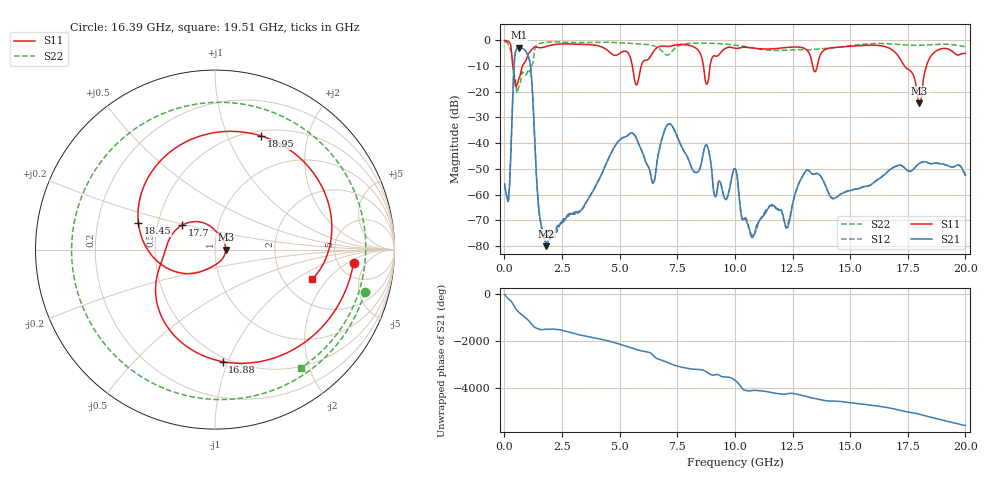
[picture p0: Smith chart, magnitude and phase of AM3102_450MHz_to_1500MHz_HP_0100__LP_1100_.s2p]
!Agilent Technologies,E8364B,MY43040894,A.07.50.67
!Agilent E8364B: A.07.50.67
!Date: Thursday, January 11, 2018 05:38:16
!Correction: S11(Full 2 Port(1,2))
!S21(Full 2 Port(1,2))
!S12(Full 2 Port(1,2))
!S22(Full 2 Port(1,2))
!S2P File: Measurements: S11, S21, S12, S22:
# Hz S  dB  R 50
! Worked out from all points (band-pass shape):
!   1601 points, 10 MHz to 20 GHz, reference 50 ohm
!   highest |S21| = -2.88 dB at 634.7 MHz (marker M1); lowest = -80.1 dB at 1.822 GHz (marker M2)
!   |S21| within 3 dB of the highest: 459.8 MHz to 1.021 GHz (560.8 MHz wide, 75.8 % of centre)
!   lowest |S11| = -24.5 dB at 18 GHz (marker M3), VSWR 1.13, Z = 56.4 + j0.00754 ohm
!   |S11| at or under -10 dB: 366.2 MHz to 781.8 MHz (415.5 MHz wide, 72.4 % of centre); 5.551 GHz to 5.938 GHz (387.2 MHz wide, 6.74 % of centre); 17.36 GHz to 18.31 GHz (951.1 MHz wide, 5.33 % of centre)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
!   |S22| runs from -20.5 to -0.5 dB; largest |S21 - S12| = 0.0025
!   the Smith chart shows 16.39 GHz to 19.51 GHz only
!   S11 on the Smith chart (normalised r, x): 16.39 GHz: 6.96, -2.54; 16.88 GHz: 0.47, -0.96; 17.7 GHz: 0.67, +0.19; 18.45 GHz: 0.39, +0.14; 18.95 GHz: 0.56, +1.33; 19.51 GHz: 2.88, -1.39
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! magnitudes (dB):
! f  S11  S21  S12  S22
! 10 MHz  -0.1  -55.8  -56.2  -0.5
! 184.9 MHz  -0.6  -61.4  -61.2  -2.0
! 447.3 MHz  -15.8  -7.0  -7.0  -14.0
! 634.7 MHz  -14.8  -2.9  -2.9  -17.9
! 1.109 GHz  -4.5  -8.7  -8.7  -12.3
! 1.497 GHz  -2.9  -66.0  -65.9  -1.3
! 1.822 GHz  -2.4  -80.1  -75.8  -0.8
! 3.346 GHz  -1.6  -65.9  -66.3  -0.9
! 5.07 GHz  -4.7  -38.2  -38.2  -1.0
! 6.682 GHz  -2.6  -44.2  -44.2  -3.0
! 10.01 GHz  -3.1  -50.0  -49.9  -1.9
! 10.77 GHz  -3.0  -76.5  -76.0  -3.0
! 13.34 GHz  -8.6  -52.0  -51.9  -3.6
! 16.39 GHz  -2.2  -53.1  -52.9  -1.2
! 16.68 GHz  -3.0  -50.7  -50.7  -1.3
! 16.88 GHz  -4.1  -49.5  -49.4  -1.5
! 17.7 GHz  -12.8  -50.5  -50.5  -1.9
! 18 GHz  -24.5  -47.9  -47.9  -1.9
! 18.45 GHz  -6.9  -47.9  -47.9  -1.8
! 18.95 GHz  -3.3  -48.1  -48.1  -1.5
! 19.51 GHz  -4.9  -49.2  -49.1  -1.8
! 20 GHz  -5.1  -52.5  -52.7  -2.4
